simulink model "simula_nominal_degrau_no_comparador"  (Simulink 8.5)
settings: Solver=ode45  StartTime=0.0  StopTime=tf  RelTol=1e-3
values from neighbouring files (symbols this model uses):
  denK = [1/6 1]    [princi_JL_incerto_prefilt_2a_ordem.m]
  knom = r*kT/Ra/Jeq    [princi_JL_incerto_prefilt_2a_ordem.m]
  numK = 2.5    [princi_JL_incerto_prefilt_2a_ordem.m]
  pnom = feq/Jeq    [princi_JL_incerto_prefilt_2a_ordem.m]

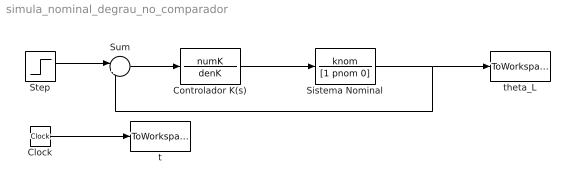
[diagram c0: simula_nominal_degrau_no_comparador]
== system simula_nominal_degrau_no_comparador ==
  Clock : Clock
  Controlador K(s) : TransferFcn  Numerator=numK  Denominator=denK
  Sistema Nominal : TransferFcn  Numerator=knom  Denominator=[1 pnom 0]
  Step : Step  Time=0  SampleTime=0
  Sum : Sum  Inputs=|+-
  t : ToWorkspace  VariableName=t  SampleTime=-1
  theta_L : ToWorkspace  VariableName=theta_L_nom  SampleTime=-1
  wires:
  Sum/1 -> Controlador K(s)/1
  Clock/1 -> t/1
  Controlador K(s)/1 -> Sistema Nominal/1
  Sistema Nominal/1 -> Sum/2, theta_L/1
  Step/1 -> Sum/1
